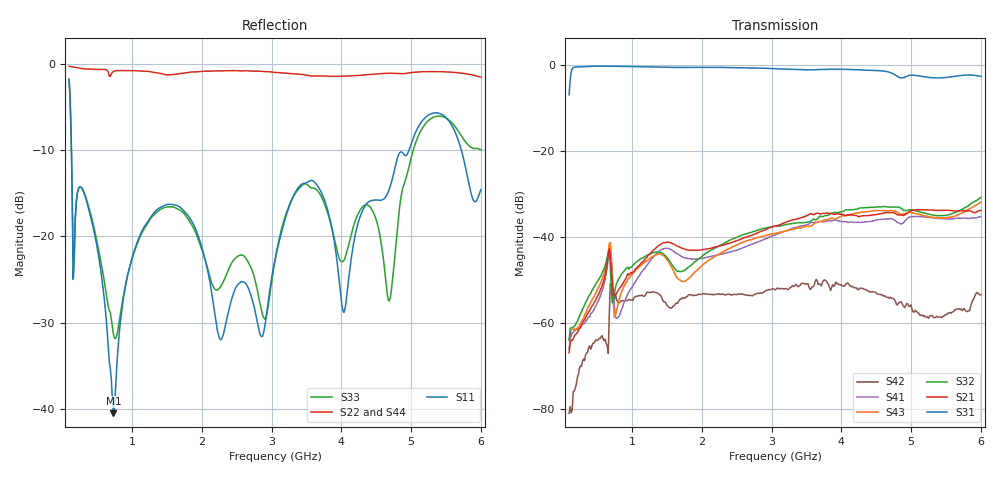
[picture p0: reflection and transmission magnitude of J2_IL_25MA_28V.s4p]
!Keysight Technologies,N5242B,MY61256241,Z.15.82.127
!Date: Friday, August 25, 2023 02:20:25
!Correction: S11(C  4-Port  )
!S12(C  4-Port  )
!S13(C  4-Port  )
!S14(C  4-Port  )
!S21(C  4-Port  )
!S22(C  4-Port  )
!S23(C  4-Port  )
!S24(C  4-Port  )
!S31(C  4-Port  )
!S32(C  4-Port  )
!S33(C  4-Port  )
!S34(C  4-Port  )
!S41(C  4-Port  )
!S42(C  4-Port  )
!S43(C  4-Port  )
!S44(C  4-Port  )
!S4P File: Measurements: <S11,S12,S13,S14>,
!<S21,S22,S23,S24>,
!<S31,S32,S33,S34>,
!<S41,S42,S43,S44>:
# Hz S  dB  R 50
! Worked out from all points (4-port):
!   401 points, 100 MHz to 6 GHz, reference 50 ohm
!   strongest paths, dB at 100 MHz, 1.575 GHz, 3.05 GHz, 4.525 GHz, 6 GHz:
!     S31: -7.0, -0.7, -1.0, -1.4, -2.7
!     S21: -67.0, -41.5, -37.5, -34.8, -33.9
!     S32: -64.1, -46.5, -37.6, -33.1, -30.9
!     S43: -63.9, -47.3, -39.3, -33.9, -32.0
!     S41: -66.2, -43.1, -39.6, -36.1, -35.3
!     S42: -81.0, -56.5, -52.3, -53.4, -53.5
!   lowest |S11| = -40.5 dB at 734.2 MHz (marker M1), VSWR 1.02, Z = 49.3 - j0.592 ohm
!   |S11| at or under -10 dB: 133.1 MHz to 4.969 GHz (4.836 GHz wide, 190 % of centre); 5.72 GHz to end of sweep
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1e8  -1.78 -106.2  -67.24 159.7  -7.04 154.2  -66.09 168.6
     -66.98 161.4  -0.26 -72.6  -63.84 172.7  -79.58 -123.9
     -7.03 154.2  -64.11 171.7  -1.79 -106.6  -63.82 174.4
     -66.19 168.1  -81.04 -122.3  -63.90 176.5  -0.28 -72.9
7.3425e8  -40.50 -140.5  -53.10 73.2  -0.39 -142.3  -52.84 34.0
          -53.15 72.4  -0.89 81.0  -54.24 -44.9  -53.55 9.0
          -0.39 -142.3  -54.29 -44.5  -31.30 -157.2  -55.57 -131.2
          -52.87 34.7  -53.53 9.4  -55.57 -131.3  -0.90 80.7
1.67825e9  -16.55 95.7  -42.38 -133.9  -0.67 0.1  -44.23 -134.3
           -42.38 -134.0  -1.13 -104.5  -48.10 127.0  -54.85 170.7
           -0.66 0.1  -48.10 126.4  -16.91 75.8  -49.98 104.1
           -44.24 -134.4  -54.80 170.9  -49.97 103.8  -1.17 -103.7
2.65175e9  -25.72 54.6  -40.01 61.5  -0.77 142.3  -42.16 66.1
           -39.99 61.4  -0.79 91.3  -39.28 -40.9  -53.51 -3.7
           -0.77 142.4  -39.26 -40.8  -22.77 88.3  -40.93 -44.5
           -42.16 66.2  -53.56 -4.0  -40.91 -44.4  -0.83 92.1
3.286e9  -15.82 79.7  -36.15 -59.2  -1.09 1.1  -38.13 -52.1
         -36.16 -59.1  -1.11 -12.7  -36.99 -165.7  -51.87 -107.6
         -1.09 1.1  -36.98 -165.6  -15.80 88.4  -38.34 -171.1
         -38.14 -52.1  -51.66 -107.5  -38.34 -170.9  -1.12 -10.8
4.12675e9  -23.55 128.3  -34.94 126.5  -1.14 172.9  -36.60 135.6
           -34.95 126.5  -1.39 -176.4  -33.73 22.1  -51.41 88.3
           -1.14 173.0  -33.72 22.2  -20.30 32.9  -34.77 17.8
           -36.60 135.6  -51.43 88.2  -34.79 17.8  -1.41 -173.6
6e9  -14.57 73.3  -33.95 146.4  -2.70 114.6  -35.35 154.0
     -33.93 146.4  -1.54 -99.3  -30.89 9.0  -53.55 173.9
     -2.69 114.7  -30.89 9.1  -9.95 -47.0  -31.99 6.1
     -35.35 154.2  -53.50 174.0  -32.02 6.1  -1.51 -97.6
